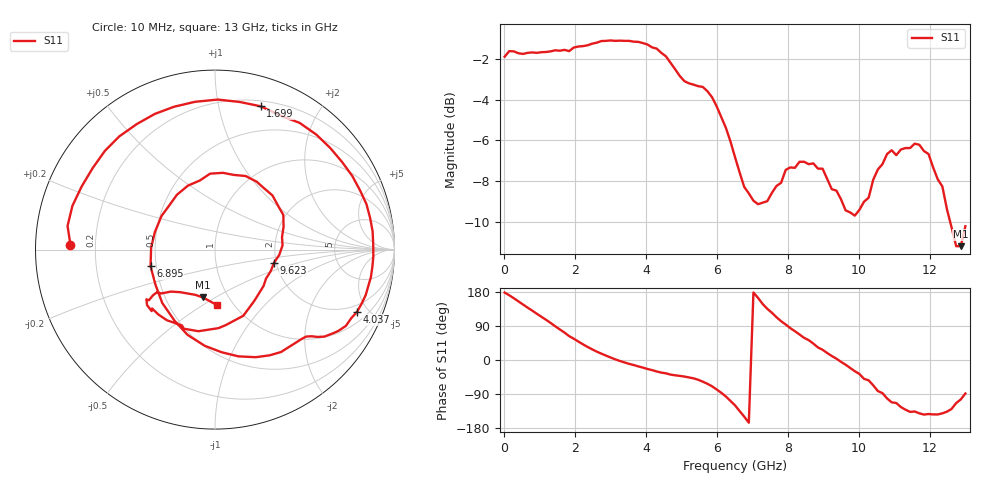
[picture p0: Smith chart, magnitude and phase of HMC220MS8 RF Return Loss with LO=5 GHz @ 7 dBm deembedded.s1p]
!Hittite Microwave Corporation
!12 Elizabeth Drive
!Chelmsford, MA 01824
!Tel: 978-250-3343
!Fax: 978-250-3373
!Device: HMC220MS8, 5-12 GHz, GaAS MMIC SMT Double-Balanced Mixer in 8-lead MSOP package
!Misc: RF Return Loss, LO = 5 GHz @ 7dBm, Room
# MHZ S MA R 50
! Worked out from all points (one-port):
!   101 points, 10 MHz to 13 GHz, reference 50 ohm
!   lowest |S11| = -11.2 dB at 12.87 GHz (marker M1), VSWR 1.76, Z = 38.2 - j22.1 ohm
!   |S11| at or under -10 dB: 12.57 GHz to end of sweep
!   S11 on the Smith chart (normalised r, x): 10 MHz: 0.11, +0.02; 1.699 GHz: 0.25, +1.34; 4.037 GHz: 1.55, -4.23; 6.895 GHz: 0.46, -0.10; 9.623 GHz: 1.95, -0.32; 13 GHz: 0.84, -0.57
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10  0.806 178.0
399.7  0.822 154.7
919.3  0.824 122.0
1309  0.831 97.6
1698.7  0.838 72.3
2088.4  0.854 48.6
2478.1  0.868 28.2
3257.5  0.883 -2.5
4036.9  0.864 -23.7
4946.2  0.723 -41.9
5595.7  0.679 -57.2
5985.4  0.609 -77.6
6505  0.456 -119.6
6894.7  0.371 -165.5
7544.2  0.372 124.8
7933.9  0.424 93.7
8193.7  0.429 76.0
8973.1  0.427 27.0
9622.6  0.337 -12.4
9752.5  0.333 -21.1
10272.1  0.362 -53.6
10531.9  0.425 -81.9
10791.7  0.464 -101.5
11441.2  0.48 -136.9
11830.9  0.472 -144.1
12350.5  0.386 -140.7
12870.1  0.275 -104.0
13000  0.308 -88.4
